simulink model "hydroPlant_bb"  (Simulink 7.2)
settings: Solver=ode23tb  StartTime=0.0  StopTime=1000  MaxStep=0.5  RelTol=1e-3
undefined symbols (not defined in the file or in its folder): Hydorplant_sf, sigbuilder_block

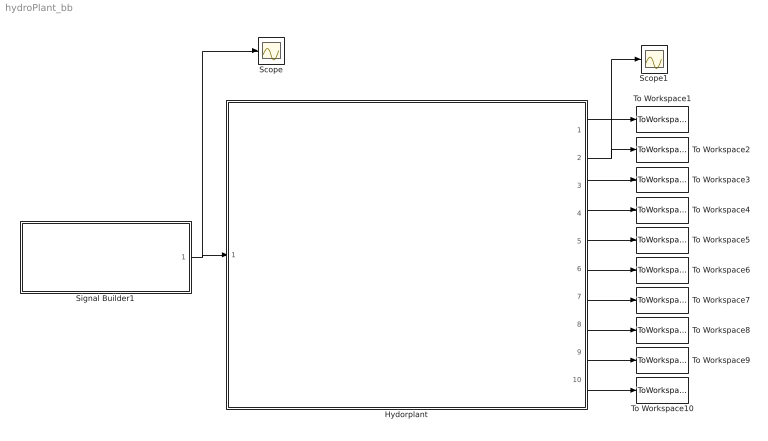
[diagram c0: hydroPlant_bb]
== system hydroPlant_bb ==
  Hydorplant : Subsystem
  Scope : Scope
  Scope1 : Scope
  Signal Builder1 : Subsystem  Tag=STV Subsys  LoadFcn=sigbuilder_block('load');  StartFcn=sigbuilder_block('start');  StopFcn=sigbuilder_block('stop');  ClipboardFcn=sigbuilder_block('clipboard');
  To Workspace1 : ToWorkspace  VariableName=time_bb  SampleTime=-1  SaveFormat=Array
  To Workspace10 : ToWorkspace  VariableName=P_bb  SampleTime=-1  SaveFormat=Array
  To Workspace2 : ToWorkspace  VariableName=x_bb  SampleTime=-1  SaveFormat=Array
  To Workspace3 : ToWorkspace  VariableName=h_W_bb  SampleTime=-1  SaveFormat=Array
  To Workspace4 : ToWorkspace  VariableName=p_F_bb  SampleTime=-1  SaveFormat=Array
  To Workspace5 : ToWorkspace  VariableName=V_flw_T_bb  SampleTime=-1  SaveFormat=Array
  To Workspace6 : ToWorkspace  VariableName=V_flw_F_bb  SampleTime=-1  SaveFormat=Array
  To Workspace7 : ToWorkspace  VariableName=omega_bb  SampleTime=-1  SaveFormat=Array
  To Workspace8 : ToWorkspace  VariableName=U_bb  SampleTime=-1  SaveFormat=Array
  To Workspace9 : ToWorkspace  VariableName=I_bb  SampleTime=-1  SaveFormat=Array
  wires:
  Hydorplant/1(time) -> To Workspace1/1
  Hydorplant/2(x) -> To Workspace2/1, Scope1/1
  Hydorplant/3(h_W) -> To Workspace3/1
  Hydorplant/4(p_F) -> To Workspace4/1
  Hydorplant/5(v_flw_T) -> To Workspace5/1
  Hydorplant/6(v_flw_F) -> To Workspace6/1
  Hydorplant/7(omega) -> To Workspace7/1
  Hydorplant/8(U) -> To Workspace8/1
  Hydorplant/9(I) -> To Workspace9/1
  Hydorplant/10(P) -> To Workspace10/1
  Signal Builder1/1(u) -> Hydorplant/1(u), Scope/1

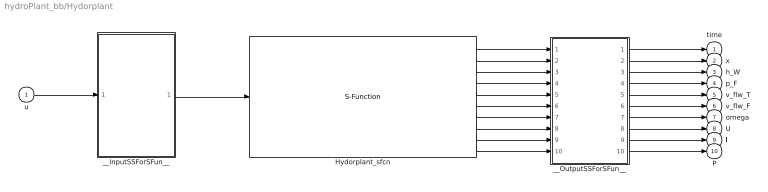
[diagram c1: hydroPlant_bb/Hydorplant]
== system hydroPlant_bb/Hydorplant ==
  u : Inport  OutDataType=sfix(16)  OutScaling=2^0
  Hydorplant_sfcn : S-Function  FunctionName=Hydorplant_sf  SFunctionModules=""  EnableBusSupport=off  mask{rtw_sf_name=Hydorplant_sf, showVar=off}
      mask prompts: rtw_sf_name "Generated S-function name (model_sf):"; showVar "Show module list"
      mask help: Real-Time Workshop generated S-function.
      mask init:
      | displist = '';
      | if ~strcmp(get_param(gcb, 'FunctionName'), rtw_sf_name);
      |   set_param(gcb, 'FunctionName', rtw_sf_name);
      | end
      | % Check if we are generating RTW code
      | rtw_mode = false;
      | if strcmpi(get_param(bdroot(gcb),'SimulationStatus'),'Initializing')
      | 	rtw_mode = strcmpi(get_param(bdroot(gcb),'BuildingRTWCode'),'on') && ...
      | 		~strcmpi(get_param(bdroot(gcb),'TargetStyle'),'SimulationTarget');
      | end
      | if showVar || rtw_mode
      | 	if exist('rtwsfunc') == 2 | exist('rtwsfunc') == 6
      | 		tmplist = rtwsfunc(rtw_sf_name,gcb);
      | 		tmplist = ['\nList of Modules:\n', tmplist];
      | 	elseif showVar
      | 		tmplist = '\nList of Modules:\nRTW not licensed\n';
      |  	end
      | end
      | if showVar
      |   displist = tmplist;
      | end
  __InputSSForSFun__ : Subsystem
  __OutputSSForSFun__ : Subsystem
  time : Outport  PortDimensions=1  SampleTime=[-1 0]  DataType=double  OutDataType=sfix(16)  OutScaling=2^0  OutDataTypeStr=double
  x : Outport  Port=2  PortDimensions=1  SampleTime=[-1 0]  DataType=double  OutDataType=sfix(16)  OutScaling=2^0  OutDataTypeStr=double
  h_W : Outport  Port=3  PortDimensions=1  SampleTime=[-1 0]  DataType=double  OutDataType=sfix(16)  OutScaling=2^0  OutDataTypeStr=double
  p_F : Outport  Port=4  PortDimensions=1  SampleTime=[-1 0]  DataType=double  OutDataType=sfix(16)  OutScaling=2^0  OutDataTypeStr=double
  v_flw_T : Outport  Port=5  PortDimensions=1  SampleTime=[-1 0]  DataType=double  OutDataType=sfix(16)  OutScaling=2^0  OutDataTypeStr=double
  v_flw_F : Outport  Port=6  PortDimensions=1  SampleTime=[-1 0]  DataType=double  OutDataType=sfix(16)  OutScaling=2^0  OutDataTypeStr=double
  omega : Outport  Port=7  PortDimensions=1  SampleTime=[-1 0]  DataType=double  OutDataType=sfix(16)  OutScaling=2^0  OutDataTypeStr=double
  U : Outport  Port=8  PortDimensions=1  SampleTime=[-1 0]  DataType=double  OutDataType=sfix(16)  OutScaling=2^0  OutDataTypeStr=double
  I : Outport  Port=9  PortDimensions=1  SampleTime=[-1 0]  DataType=double  OutDataType=sfix(16)  OutScaling=2^0  OutDataTypeStr=double
  P : Outport  Port=10  PortDimensions=1  SampleTime=[-1 0]  DataType=double  OutDataType=sfix(16)  OutScaling=2^0  OutDataTypeStr=double
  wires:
  u/1 -> __InputSSForSFun__/1(u)
  __InputSSForSFun__/1(__UniqueOutportName__1__) -> Hydorplant_sfcn/1
  Hydorplant_sfcn/1 -> __OutputSSForSFun__/1(__UniqueInportName__1__)
  Hydorplant_sfcn/2 -> __OutputSSForSFun__/2(__UniqueInportName__2__)
  Hydorplant_sfcn/3 -> __OutputSSForSFun__/3(__UniqueInportName__3__)
  Hydorplant_sfcn/4 -> __OutputSSForSFun__/4(__UniqueInportName__4__)
  Hydorplant_sfcn/5 -> __OutputSSForSFun__/5(__UniqueInportName__5__)
  Hydorplant_sfcn/6 -> __OutputSSForSFun__/6(__UniqueInportName__6__)
  Hydorplant_sfcn/7 -> __OutputSSForSFun__/7(__UniqueInportName__7__)
  Hydorplant_sfcn/8 -> __OutputSSForSFun__/8(__UniqueInportName__8__)
  Hydorplant_sfcn/9 -> __OutputSSForSFun__/9(__UniqueInportName__9__)
  Hydorplant_sfcn/10 -> __OutputSSForSFun__/10(__UniqueInportName__10__)
  __OutputSSForSFun__/1(time) -> time/1
  __OutputSSForSFun__/2(x) -> x/1
  __OutputSSForSFun__/3(h_W) -> h_W/1
  __OutputSSForSFun__/4(p_F) -> p_F/1
  __OutputSSForSFun__/5(v_flw_T) -> v_flw_T/1
  __OutputSSForSFun__/6(v_flw_F) -> v_flw_F/1
  __OutputSSForSFun__/7(omega) -> omega/1
  __OutputSSForSFun__/8(U) -> U/1
  __OutputSSForSFun__/9(I) -> I/1
  __OutputSSForSFun__/10(P) -> P/1

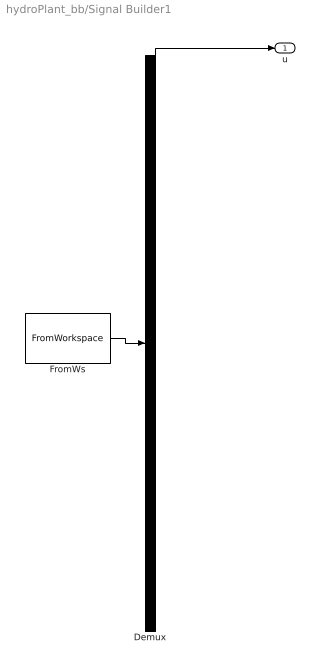
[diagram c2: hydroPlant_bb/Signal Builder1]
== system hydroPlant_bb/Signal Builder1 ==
  Demux : Demux  Tag=STV Demux  Outputs=1
  FromWs : FromWorkspace  Tag=STV FromWs  VariableName=tuvar  SampleTime=0  SigBuilderData=DataTag0  VnvData=DataTag1
  u : Outport  Tag=STV Outport
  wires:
  FromWs/1 -> Demux/1
  Demux/1 -> u/1

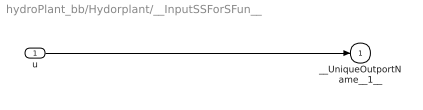
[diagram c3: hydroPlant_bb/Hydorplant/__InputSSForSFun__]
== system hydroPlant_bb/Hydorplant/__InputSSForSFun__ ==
  u : Inport  OutDataType=sfix(16)  OutScaling=2^0
  __UniqueOutportName__1__ : Outport  OutDataType=sfix(16)  OutScaling=2^0
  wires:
  u/1 -> __UniqueOutportName__1__/1

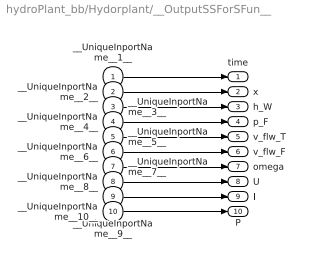
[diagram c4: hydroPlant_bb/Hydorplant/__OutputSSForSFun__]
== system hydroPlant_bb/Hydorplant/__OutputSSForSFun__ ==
  __UniqueInportName__1__ : Inport  OutDataType=sfix(16)  OutScaling=2^0
  __UniqueInportName__2__ : Inport  Port=2  OutDataType=sfix(16)  OutScaling=2^0
  __UniqueInportName__3__ : Inport  Port=3  OutDataType=sfix(16)  OutScaling=2^0
  __UniqueInportName__4__ : Inport  Port=4  OutDataType=sfix(16)  OutScaling=2^0
  __UniqueInportName__5__ : Inport  Port=5  OutDataType=sfix(16)  OutScaling=2^0
  __UniqueInportName__6__ : Inport  Port=6  OutDataType=sfix(16)  OutScaling=2^0
  __UniqueInportName__7__ : Inport  Port=7  OutDataType=sfix(16)  OutScaling=2^0
  __UniqueInportName__8__ : Inport  Port=8  OutDataType=sfix(16)  OutScaling=2^0
  __UniqueInportName__9__ : Inport  Port=9  OutDataType=sfix(16)  OutScaling=2^0
  __UniqueInportName__10__ : Inport  Port=10  OutDataType=sfix(16)  OutScaling=2^0
  time : Outport  PortDimensions=1  SampleTime=[-1 0]  DataType=double  OutDataType=sfix(16)  OutScaling=2^0  OutDataTypeStr=double
  x : Outport  Port=2  PortDimensions=1  SampleTime=[-1 0]  DataType=double  OutDataType=sfix(16)  OutScaling=2^0  OutDataTypeStr=double
  h_W : Outport  Port=3  PortDimensions=1  SampleTime=[-1 0]  DataType=double  OutDataType=sfix(16)  OutScaling=2^0  OutDataTypeStr=double
  p_F : Outport  Port=4  PortDimensions=1  SampleTime=[-1 0]  DataType=double  OutDataType=sfix(16)  OutScaling=2^0  OutDataTypeStr=double
  v_flw_T : Outport  Port=5  PortDimensions=1  SampleTime=[-1 0]  DataType=double  OutDataType=sfix(16)  OutScaling=2^0  OutDataTypeStr=double
  v_flw_F : Outport  Port=6  PortDimensions=1  SampleTime=[-1 0]  DataType=double  OutDataType=sfix(16)  OutScaling=2^0  OutDataTypeStr=double
  omega : Outport  Port=7  PortDimensions=1  SampleTime=[-1 0]  DataType=double  OutDataType=sfix(16)  OutScaling=2^0  OutDataTypeStr=double
  U : Outport  Port=8  PortDimensions=1  SampleTime=[-1 0]  DataType=double  OutDataType=sfix(16)  OutScaling=2^0  OutDataTypeStr=double
  I : Outport  Port=9  PortDimensions=1  SampleTime=[-1 0]  DataType=double  OutDataType=sfix(16)  OutScaling=2^0  OutDataTypeStr=double
  P : Outport  Port=10  PortDimensions=1  SampleTime=[-1 0]  DataType=double  OutDataType=sfix(16)  OutScaling=2^0  OutDataTypeStr=double
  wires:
  __UniqueInportName__1__/1 -> time/1
  __UniqueInportName__2__/1 -> x/1
  __UniqueInportName__3__/1 -> h_W/1
  __UniqueInportName__4__/1 -> p_F/1
  __UniqueInportName__5__/1 -> v_flw_T/1
  __UniqueInportName__6__/1 -> v_flw_F/1
  __UniqueInportName__7__/1 -> omega/1
  __UniqueInportName__8__/1 -> U/1
  __UniqueInportName__9__/1 -> I/1
  __UniqueInportName__10__/1 -> P/1
